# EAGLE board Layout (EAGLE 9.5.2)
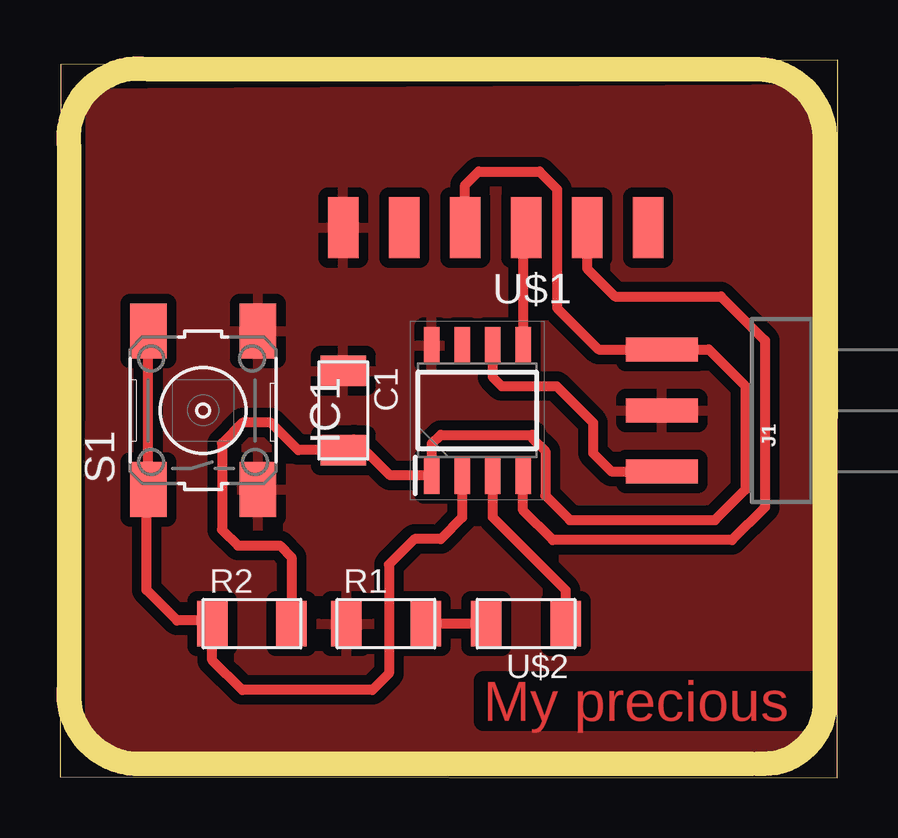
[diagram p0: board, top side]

Size 32.44 x 29.93 mm. Coordinates in mm from the lower left corner, seen from the top.
Outline: 32.41,0 32.44,29.93 0.03,29.72 0,0.05 32.41,0
Copper layers (1*16): Top 0.035mm / dielectric 1.5mm / Bottom 0.035mm
Design rules "default *": minimum track width 6mil, minimum drill 0.35mm, track to track 16mil, track to pad 16mil, pad to pad 16mil, via to via 16mil, smd to smd 16mil, copper to edge 40mil, drill to drill 6mil, minimum pad ring 10mil, minimum via ring 8mil, stop-mask expansion 4mil, vias tented up to drill 0mil, thermal gap 16mil
Milling: 11 lines

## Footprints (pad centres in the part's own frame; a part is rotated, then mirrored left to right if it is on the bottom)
C1206FAB = smd 1.27 x 1.905: 1 -1.651,0; 2 1.651,0
SOIC127P600X175-8N = smd 1.525 x 0.65: 1 -2.712,1.905; 2 -2.712,0.635; 3 -2.712,-0.635; 4 -2.712,-1.905; 5 2.712,-1.905; 6 2.712,-0.635; 7 2.712,0.635; 8 2.712,1.905
1X03_SMD_RA_MALE = smd 1 x 3: 1 -2.54,5; 2 0,5; 3 2.54,5
R1206FAB = smd 1.27 x 1.905: 1 -1.651,0; 2 1.651,0
6MM_SWITCH = smd 2.286 x 1.524: 1 -3.302,2.286; 2 3.302,2.286; 3 -3.302,-2.286; 4 3.302,-2.286
1X06SMD = smd 2.54 x 1.27: 1 0,6.35; 2 0,3.81; 3 0,1.27; 4 0,-1.27; 5 0,-3.81; 6 0,-6.35
LED1206FAB = smd 1.27 x 1.905: 1 -1.651,0; 2 1.651,0

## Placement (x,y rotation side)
C1  1  [C1206FAB]  11.81,15.32 270 top
IC1  ATTINY412-SSF  [SOIC127P600X175-8N]  17.4,15.32 90 top
J1  [1X03_SMD_RA_MALE]  30.1,15.32 90 top
R1  499  [R1206FAB]  13.59,6.43 0 top
R2  10k  [R1206FAB]  8,6.43 0 top
S1  [6MM_SWITCH]  5.97,15.32 90 top
U$1  CONN_06_FTDI-SMD-HEADER  [1X06SMD]  18.16,22.94 90 top
U$2  LEDFAB1206  [LED1206FAB]  19.43,6.43 180 top

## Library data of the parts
C1 R1 R2 S1 U$1 U$2 = fab
IC1 = ATTINY412-SSF; DESCRIPTION: 8-bit Microcontrollers - MCU 20MHz, 4KB, SOIC8, Ind 125C, Green, Tube; HEIGHT: 1.75mm; MANUFACTURER_NAME: Microchip; MANUFACTURER_PART_NUMBER: ATTINY412-SSF; MOUSER_PART_NUMBER: 579-ATTINY412-SSF; MOUSER_PRICE-STOCK: https://www.mouser.com/Search/Refine.aspx?Keyword=579-ATTINY412-SSF
J1 = SparkFun-Connectors; PROD_ID: CONN-10925

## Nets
GND: C1.1 IC1.8 J1.2 R1.1 S1.3 S1.4 U$1.1
N$1: IC1.3 U$2.1
N$2: IC1.4 U$1.5
N$3: IC1.5 U$1.4
N$4: IC1.2 R2.1 S1.1 S1.2
N$6: R1.2 U$2.2
N$7: IC1.6 J1.1
VCC: C1.2 IC1.1 J1.3 R2.2 U$1.3

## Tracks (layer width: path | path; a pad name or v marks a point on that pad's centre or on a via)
GND
  pour Top: 0.13,0.08 0.13,30.05 32.64,30.05 32.64,0.08
N$1
  Top 0.406: IC1.3 18.03,10.87 21.08,7.82 U$2.1
N$2
  Top 0.406: U$1.5 21.97,21.23 23.14,20.07 27.56,20.07 29.39,18.24 29.39,11.28 28.02,9.91 20.55,9.91 19.3,11.15 IC1.4
N$3
  Top 0.406: U$1.4 19.3,22.81 IC1.5
N$4
  Top 0.406: IC1.2 16.76,10.85 15.88,9.96 14.78,9.96 13.72,8.89 13.72,4.34 13.03,3.66 7.6,3.66 6.35,4.9 R2.1 6.22,6.55 4.88,6.55 3.61,7.82 3.61,11.94 S1.1 S1.2
N$6
  Top 0.406: U$2.2 R1.2
N$7
  Top 0.406: IC1.6 18.03,16.71 18.42,16.33 20.7,16.33 22.23,14.81 22.23,13.54 22.99,12.78 J1.1
VCC
  Top 0.406: U$1.3 16.89,24.71 17.45,25.27 19.99,25.27 20.73,24.54 20.73,19.58 22.45,17.86 J1.3 27.05,17.86 28.58,16.33 28.58,12.01 27.31,10.74 21.26,10.74 20.24,11.76 20.24,13.62 19.69,14.17 19.69,14.3 15.88,14.3 15.49,13.92 IC1.1 13.76,12.6 12.26,14.11 C1.2 9.93,13.67 8.79,14.81 7.62,14.81 6.76,13.94 6.76,10.34 7.42,9.68 9.17,9.68 9.65,9.2 R2.2

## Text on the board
Top: My precious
